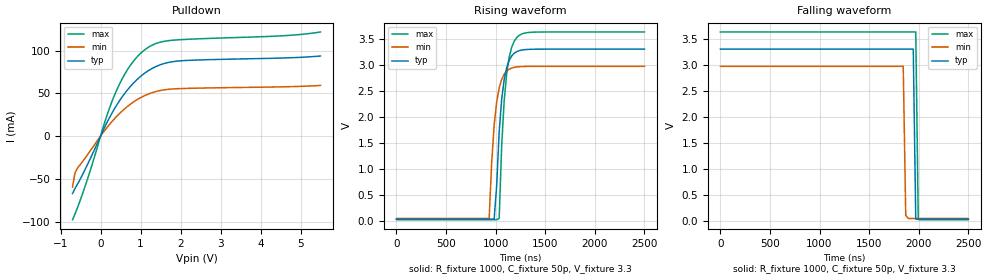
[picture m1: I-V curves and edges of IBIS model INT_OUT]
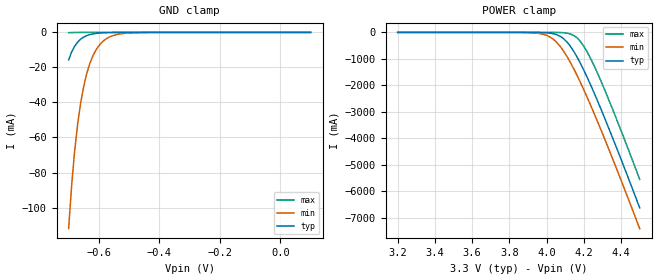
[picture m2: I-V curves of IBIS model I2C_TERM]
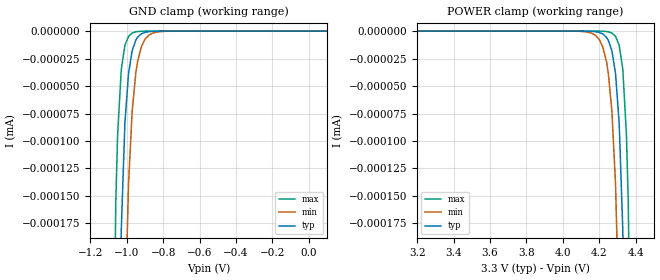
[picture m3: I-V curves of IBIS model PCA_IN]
|   NXP Semiconductors Inc.
|   Specialty Logic Products Group
|   IBIS model of PCA9544A
|   4-Channel I2C switch with
|   interrupt logic
[IBIS Ver]   3.2
[Comment Char]   |_char
| VDD typ = 3.3V, min = 2.97V and max = 3.63V
[File name]   pca9544a_3_3v.ibs
[File Rev]   1.0
[Date]   Nov 29, 2007 11:15:22 AM
[Source]
Generated by Seshadri Venkataramanan with IbisToolKit at Tempe, AZ
[Notes]
[Disclaimer]
* All rights reserved
NXP Semiconductors warrants and represents that the IBIS models identified
herein are owned by NXP Semiconductors (NXP). The
models provided are not warranted as fully representing all of the operating
characteristics and specifications of the semiconductor products to which the
models relate. Moreover, unless there is a
signed, written agreement to the contrary, these models are furnished on an "as
is" basis without support or warranty of any kind, either expressed or implied,
regarding the use thereof, and NXP specifically disclaims all implied warranties
of merchantability and
fitness of the models for any purpose.
NXP does not assume any liability arising out of the application or use of these
IBIS models including infringement of patents and
copyrights, nor does NXP convey any license under its patents and copyrights or
the rights of others.
NXP provides IBIS models as a service to our customers. You and your company
shall not distribute, convey, sell, or give these models
to anyone else without receiving prior written permission from NXP.(C) Copyright
2007 NXP Semiconductors
NXP Semiconductors (NXP) does not warrant that this model and any other
accompanying information (Model) accurately or fully represents the
operating characteristics and specifications of the semiconductor
products to which the Model relates.  Moreover, the Model is furnished
on an "as is" and with "all faults" basis, and without support or
warranty of any kind.  NXP disclaims all warranties, whether expressed
or implied or statutory, including without limitation all implied
warranties of non-infringement, merchantability and fitness for any
purpose, and those arising from a course of dealing or usage of trade.
NXP does not convey any license under its or any third party's patents,
copyrights or other intellectual property or proprietary rights.
You and your company assume any and all risks and liability arising out
of the application or use of the Model.
In no event shall NXP be liable for any direct, indirect, special,
consequential or incidental damages, however caused, whether in
warranty, contract or tort (including negligence), strict liability or
other legal theory, including, without limitation, for lost profits,
business interruption, or corruption or loss of data or information,
arising out of or in connection with the use of or the inability to use
the Model, even if NXP has been advised of the possibility of such
damages.
NXP provides the Model as a courtesy to our customers. You and your
company shall not distribute, convey, sell, or give the Model to anyone
else without receiving prior written permission from NXP.
NXP reserves the right to make changes without notice to the Model to
improve reliability, function, or design.
Please be aware that your receipt and subsequent use of the Model shall
serve as acceptance of these terms and conditions.  If you do not
accept these terms, return or destroy the Model immediately.
[Copyright]
2007
[Component]   PCA9544AD
Si_location Pin
Timing_location Pin
[Manufacturer]   NXP Semiconductors
[Package]
|   variable   typ   min   max
R_pkg   5.95E-02   5.36E-02   6.59E-02
L_pkg   4.21E-09   3.07E-09   5.91E-09
C_pkg   0.910E-12   0.758E-12   1.110E-12
|   SO20
[Pin] signal_name   model_name   R_pin   L_pin   C_pin
1   A0   PCA_IN   5.75E-02  5.91E-09  1.050E-12
2   A1   PCA_IN   6.25E-02  4.85E-09  1.040E-12
3   a2   PCA_IN   6.59E-02  3.92E-09  0.861E-12
4   INT0B   INT_IN   5.79E-02  3.32E-09  0.803E-12
5   SD0   I2C_TERM   5.36E-02  3.07E-09  0.758E-12
6   SC0   I2C_TERM   5.36E-02  3.07E-09  0.758E-12
7   INT1B   INT_IN   5.79E-02  3.32E-09  0.803E-12
8   SD1   I2C_TERM   6.59E-02  3.92E-09  0.861E-12
9   SC1   I2C_TERM   6.25E-02  4.85E-09  1.040E-12
10   Vss   GND   5.75E-02  5.91E-09  1.110E-12
11   INT2B   INT_IN   5.75E-02  5.91E-09  1.110E-12
12   SD2   I2C_TERM   6.25E-02  4.85E-09  1.040E-12
13   SC2   I2C_TERM   6.59E-02  3.92E-09  0.861E-12
14   INT3B   INT_IN   5.79E-02  3.32E-09  0.803E-12
15   SD3   I2C_TERM   5.36E-02  3.07E-09  0.758E-12
16   SC3   I2C_TERM   5.36E-02  3.07E-09  0.758E-12
17   INTB   INT_OUT   5.79E-02  3.32E-09  0.803E-12
18   SCL   I2C_TERM   6.59E-02  3.92E-09  0.861E-12
19   SDA   I2C_TERM   6.25E-02  4.85E-09  1.040E-12
20   Vdd   POWER   5.75E-02  5.91E-09  1.110E-12
[Component]   PCA9544APW
Si_location Pin
Timing_location Pin
[Manufacturer]   NXP Semiconductors
[Package]
|   variable   typ   min   max
R_pkg   7.24E-02   6.63E-02   8.34E-02
L_pkg   2.47E-09   2.09E-09   3.18E-09
C_pkg   0.341E-12   0.282E-12   0.420E-12
|   TSSOP20
[Pin] signal_name   model_name   R_pin   L_pin   C_pin
1   A0   PCA_IN   6.63E-02  3.18E-09  0.408E-12
2   A1   PCA_IN   6.67E-02  2.55E-09  0.398E-12
3   A2   PCA_IN   8.34E-02  2.35E-09  0.317E-12
4   INT0B   INT_IN   7.44E-02  2.16E-09  0.293E-12
5   SD0   I2C_TERM   7.10E-02  2.09E-09  0.282E-12
6   SC0   I2C_TERM   7.10E-02  2.09E-09  0.282E-12
7   INT1B   INT_IN   7.44E-02  2.16E-09  0.293E-12
8   SD1   I2C_TERM   8.34E-02  2.35E-09  0.317E-12
9   SC1   I2C_TERM   6.67E-02  2.55E-09  0.397E-12
10   Vss   GND   6.63E-02  3.18E-09  0.420E-12
11   INT2B   INT_IN   6.63E-02  3.17E-09  0.420E-12
12   SD2   I2C_TERM   6.67E-02  2.55E-09  0.397E-12
13   SC2   I2C_TERM   8.34E-02  2.35E-09  0.317E-12
14   INT3B   INT_IN   7.44E-02  2.16E-09  0.293E-12
15   SD3   I2C_TERM   7.10E-02  2.09E-09  0.282E-12
16   SC3   I2C_TERM   7.10E-02  2.09E-09  0.282E-12
17   INTB   INT_OUT   7.44E-02  2.16E-09  0.293E-12
18   SCL   I2C_TERM   8.34E-02  2.35E-09  0.317E-12
19   SDA   I2C_TERM   6.67E-02  2.55E-09  0.398E-12
20   Vdd   POWER   6.63E-02  3.17E-09  0.420E-12
[Component]   PCA9544ABS
Si_location Pin
Timing_location Pin
[Manufacturer]   NXP Semiconductors
[Package]
|   variable   typ   min   max
R_pkg   0.364   0.215   0.513
L_pkg   1.49E-09   1.04E-09   1.93E-09
C_pkg   0.149E-12   0.124E-12   0.173E-12
|   HVQFN20
[Package Model]   hvqfn20
[Pin] signal_name   model_name
1   A2   PCA_IN
2   INT0B   INT_IN
3   SD0   I2C_TERM
4   SC0   I2C_TERM
5   INT1B   INT_IN
6   SD1   I2C_TERM
7   SC1   I2C_TERM
8   Vss   GND
9   INT2B   INT_IN
10   SD2   I2C_TERM
11   SC2   I2C_TERM
12   INT3B   INT_IN
13   SD3   I2C_TERM
14   SC3   I2C_TERM
15   INTB   INT_OUT
16   SCL   I2C_TERM
17   SDA   I2C_TERM
18   Vdd   POWER
19   A0   PCA_IN
20   A1   PCA_IN
[Series Pin Mapping] pin_2 model_name   function_table_group
18   6   PCA_SW   1
18   9   PCA_SW   2
18   13   PCA_SW   3
18   16   PCA_SW   4
19   5   PCA_SW   1
19   8   PCA_SW   2
19   12   PCA_SW   3
19   15   PCA_SW   4
[Series Switch Groups]
|   Function Group States
|  default
Off 1 2 3 4 /
On 1 /
On 2 /
On 3 /
On 4 /
|  [Define Package Model]  MLF20_PCA9564.pkg
[Define Package Model]   hvqfn20
[Manufacturer]   Unknown
[OEM]   Unknown
[Description]   none
[Number of Pins]   20
[Pin Numbers]
|   1 = D2
1
|   2 = D3
2
|   3 = D4
3
|   4 = D5
4
|   5 = D6
5
|   6 = D7
6
|   7 = NC
7
|   8 = Vss
8
|   9 = WRn
9
|   10 = RDn
10
|   11 = CEn
11
|   12 = A0
12
|   13 = A1
13
|   14 = INTn
14
|   15 = RESETn
15
|   16 = SCL
16
|   17 = SDA
17
|   18 = Vdd
18
|   19 = D0
19
|   20 = D1
20
[Model Data]
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[End Model Data]
[End Package Model]
[Model]   PCA_SW
Model_type Series_switch
C_comp   0   0   0
[Temperature Range] 27   85   -40
[Voltage Range]   3.3   2.97   3.63
[Pullup Reference]  3.3   2.97   3.63
[Pulldown Reference]0   0   0
[On]
[R Series]   11   5   30
[C Series]   3p   NA   5p
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[Off]
|   variable   R(typ)   R(min)   R(max)
[R Series]   1e06   1e06   1e06
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| Models and submodels in the file (5): INT_OUT (Open_drain), I2C_TERM (Terminator), PCA_IN (Input), INT_IN (Input), PCA_SW (Series_switch)
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[Model]   INT_OUT
Model_type Open_drain
Vref=3.3
Vmeas=1.65
Rref=1000
Cref=1p
C_comp   2.2p   2p   2.3p
[Model Spec]
Vmeas   1.65   1.485   1.815
[Temperature Range] 27   85   -40
[Voltage Range]   3.3   2.97   3.63
[Pullup Reference]  3.3   2.97   3.63
[Pulldown Reference]0   0   0
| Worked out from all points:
|   slope of the pulldown table from 0 to 0.495 V, typ, clamps not added: 11.6 ohm
|   falling waveform, R_fixture 1000, C_fixture 50p, V_fixture 3.3: 20-80 % time 15.2ns typ, 15.5ns min, 15.2ns max; typ from 3.3 V to 0.031 V
|   rising waveform, R_fixture 1000, C_fixture 50p, V_fixture 3.3: 20-80 % time 71ns typ, 71.3ns min, 69.6ns max; typ from 0.031 V to 3.3 V
[Pulldown]
-700mV    -67.14mA   -59.47mA   -97.7mA
-640mV    -61.24mA   -42.97mA   -91.29mA
-570mV    -55.56mA   -36.96mA   -82.89mA
-260mV    -26.66mA   -17.34mA   -40.55mA
110mV     11.11mA    7.003mA    17.12mA
360mV     32.93mA    20.97mA    49.15mA
550mV     46.52mA    29.8mA     67.88mA
740mV     57.79mA    37.16mA    82.48mA
1.12V     74.18mA    47.76mA    101.5mA
1.43V     82.31mA    52.71mA    109mA
1.93V     87.8mA     55.48mA    112.6mA
5.5V      93.73mA    59.3mA     121.8mA
[Falling Waveform]
R_fixture=1000
C_fixture=50p
V_fixture=3.3
V_fixture_min=2.97
V_fixture_max=3.63
0s        3.3V       2.97V      3.63V
1.843us   3.3V       2.97V      3.63V
1.869us   3.3V       104.3mV    3.63V
1.894us   3.3V       45.24mV    3.63V
1.944us   3.3V       45.03mV    3.63V
1.97us    33.47mV    45.03mV    3.63V
1.995us   31.49mV    45.03mV    25.52mV
2.5us     31.48mV    45.03mV    22.23mV
[Rising Waveform]
R_fixture=1000
C_fixture=50p
V_fixture=3.3
V_fixture_min=2.97
V_fixture_max=3.63
0s        31.48mV    45.02mV    22.23mV
934.3ns   31.49mV    45.31mV    22.24mV
984.8ns   31.5mV     1.838V     22.25mV
1.01us    674.2mV    2.283V     22.24mV
1.035us   1.707V     2.553V     46.47mV
1.061us   2.334V     2.717V     1.446V
1.111us   2.945V     2.877V     2.828V
1.162us   3.17V      2.936V     3.336V
1.237us   3.271V     2.962V     3.565V
2.5us     3.3V       2.97V      3.63V
[Ramp]
R_load=1000
dV/dt_r   2.157E+0/1.028E-9   2.145E+0/1.326E-9   2.165E+0/7.615E-10
dV/dt_f   2.157E+0/1.067E-9   2.145E+0/1.643E-9   2.165E+0/1.092E-9
|[End   INT_OUT
| [End   INT_OUT
|  [End   INT_OUT
[Model]   I2C_TERM
Model_type Terminator
C_comp   1.7p   1.7p   1.7p
[Temperature Range] 27   85   -40
[Voltage Range]   3.3   2.97   3.63
[Pullup Reference]  3.3   2.97   3.63
[Pulldown Reference]0   0   0
[POWER Clamp Reference]3.3   2.97   3.63
[GND Clamp Reference]0   0   0
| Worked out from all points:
|   GND clamp passes 1 mA (typ) near -0.62 V on its own axis
[GND Clamp]
|   -6.000000E-1   -1.554225E-1   -1.242642E-1   -2.666059E-1
|   -5.000000E-1   -1.602113E-1   -1.179351E-1   -2.662641E-1
|   -4.000000E-1   -1.574088E-1   -1.099432E-1   -2.800035E-1
-700mV    -15.71mA   -112mA     -166.1uA
-690mV    -11.17mA   -87.19mA   -101uA
-680mV    -7.88mA    -67.53mA   -61.45uA
-670mV    -5.512mA   -52.09mA   -37.37uA
-660mV    -3.829mA   -40.04mA   -22.72uA
-650mV    -2.644mA   -30.68mA   -13.81uA
-640mV    -1.818mA   -23.41mA   -8.398uA
-620mV    -851uA     -13.45mA   -3.104uA
-580mV    -183.1uA   -4.156mA   -424nA
-540mV    -39.09uA   -1.196mA   -57.99nA
-480mV    -3.844uA   -174.4uA   -3.016nA
100mV     19.7pA     22.78pA    19.7pA
[POWER Clamp]
3.2V      19.7pA     22.78pA    19.7pA
3.92V     -851uA     -13.45mA   -3.104uA
3.99V     -11.17mA   -87.19mA   -101uA
4.04V     -56.45mA   -282.7mA   -1.201mA
4.08V     -178.2mA   -594.7mA   -8.128mA
4.12V     -452.4mA   -1.037A    -44.8mA
4.17V     -1.013A    -1.717A    -251.3mA
4.21V     -1.576A    -2.326A    -641.4mA
4.26V     -2.362A    -3.138A    -1.332A
4.32V     -3.374A    -4.162A    -2.304A
4.39V     -4.61A     -5.399A    -3.529A
4.5V      -6.62A     -7.403A    -5.544A
[Model]   PCA_IN
Model_type Input
Vinh=2.1
Vinl=0.9
C_comp   0.5p   0.5p   0.5p
[Model Spec]
[Temperature Range] 27   85   -40
[Voltage Range]   3.3   2.97   3.63
[POWER Clamp Reference]3.3   2.97   3.63
[GND Clamp Reference]0   0   0
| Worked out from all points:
|   GND clamp passes 1 mA (typ) near -1.25 V on its own axis
[GND Clamp]
-1.7V     -4.583A    -3.655A    -5.795A
-1.08V    -1.254uA   -2.572uA   -421.3nA
-1.06V    -578.9nA   -1.345uA   -155.7nA
-1.05V    -393.3nA   -972.8nA   -94.64nA
-1.03V    -181.5nA   -508.9nA   -34.97nA
-1.01V    -83.76nA   -266.2nA   -12.93nA
-990mV    -38.66nA   -139.2nA   -4.777nA
-970mV    -17.84nA   -72.82nA   -1.766nA
-950mV    -8.234nA   -38.09nA   -653.2pA
-920mV    -2.582nA   -14.41nA   -147.4pA
-860mV    -254.6pA   -2.063nA   -8.255pA
100mV     100fA      100fA      100fA
[POWER Clamp]
3.2V      100fA      100fA      100fA
4.16V     -254.6pA   -2.063nA   -8.255pA
4.22V     -2.582nA   -14.41nA   -147.4pA
4.25V     -8.234nA   -38.09nA   -653.2pA
4.27V     -17.84nA   -72.82nA   -1.766nA
4.29V     -38.66nA   -139.2nA   -4.777nA
4.31V     -83.76nA   -266.2nA   -12.93nA
4.33V     -181.5nA   -508.9nA   -34.97nA
4.35V     -393.3nA   -972.8nA   -94.64nA
4.36V     -578.9nA   -1.345uA   -155.7nA
4.38V     -1.254uA   -2.572uA   -421.3nA
5V        -4.583A    -3.655A    -5.795A
